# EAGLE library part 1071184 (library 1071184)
PCB terminal block, nominal current: 13.5 A, rated voltage (III/2): 160 V, nominal cross section: 1.5 mm, Number of rows: 1, Number of positions per row: 7, product range: SPTA 1,5/..-THR, pitch: 3.81 mm, connection method: Push-in spring connection, mounting: THR soldering, conductor/PCB connection direction: 45 , color: black, Solder pin [P]: 2.6 mm, type of packaging: 44 mm wide tape Source: Datasheet
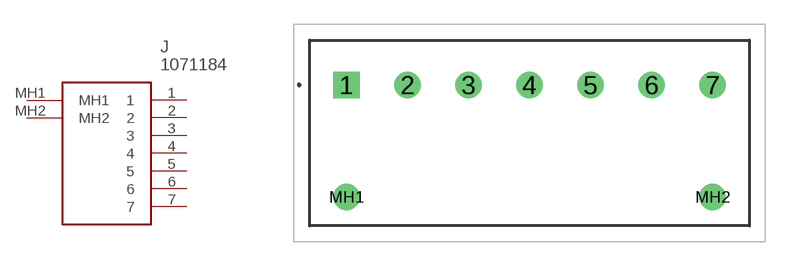
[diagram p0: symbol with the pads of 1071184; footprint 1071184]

Designator prefix J

## 1071184 (Description: PCB terminal block, nominal current: 13.5 A, rated voltage (III/2): 160 V, nominal cross section: 1.5 mm, Number of rows: 1, Number of positions per row: 7, product range: SPTA 1,5/..-THR, pitch: 3.81 mm, connection method: Push-in spring connection, mounting: THR soldering, conductor/PCB connection direction: 45 , color: black, Solder pin [P]: 2.6 mm, type of packaging: 44 mm wide tape; Height: 12.62mm; Manufacturer_Name: Phoenix Contact; Manufacturer_Part_Number: 1071184; Mouser_Part_Number: 651-1071184; Mouser_Price-Stock: https://www.mouser.co.uk/ProductDetail/Phoenix-Contact/1071184?qs=P19jvy6W2mc%252BSFHTGS8UdQ%3D%3D)  [1071184]
1  1
2  2
3  3
4  4
5  5
6  6
7  7
MH1  MH1
MH2  MH2

## Footprint 1071184 (pad centres in mm)
1071184
drill 1.1 pad 1.65 square: 1 0,0
drill 1.1 pad 1.65: 2 3.81,0; 3 7.62,0; 4 11.43,0; 5 15.24,0; 6 19.05,0; 7 22.86,0; MH1 0,-7; MH2 22.86,-7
